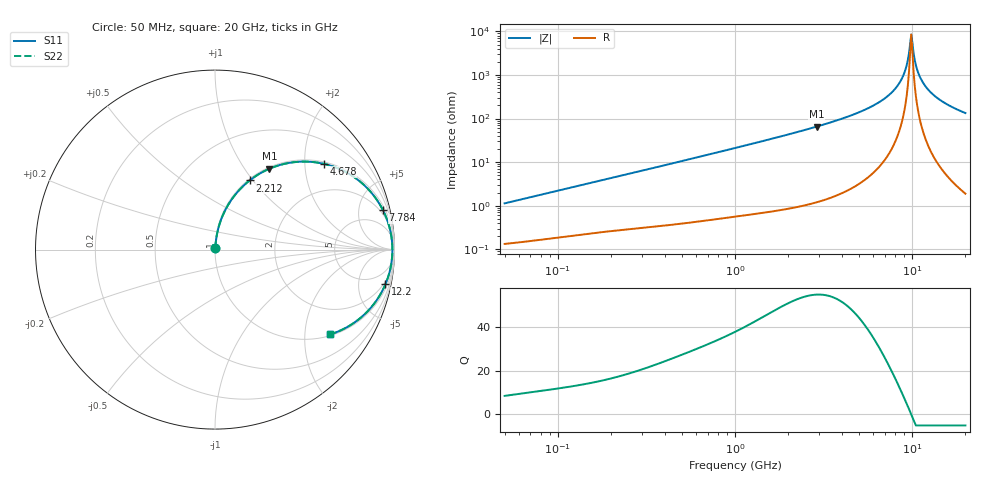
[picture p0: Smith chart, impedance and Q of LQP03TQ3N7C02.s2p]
!Murata Part Number: LQP03TQ3N7C02
!These Parameters are Measured in Series Mode Connection
!  o--[Z]--o
!Port1  Port2
!  o-------o
!Freq. Start=50[MHz] Stop=20[GHz], 401[Steps]
# Hz S RI R 50
!Freq.(Hz) S11(Real) S11(Imag) S21(Real) S21(Imag) S12(Real) S12(Imag) S22(Real) S22(Imag)
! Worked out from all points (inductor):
!   401 points, 50 MHz to 20 GHz, reference 50 ohm
!   read as one part in series: L = 3.55 nH near 51.52 MHz
!   highest Q = 54.6 at 2.896 GHz (marker M1), where L = 3.6 nH
!   self-resonance near 9.892 GHz
!   S11 on the Smith chart (normalised r, x): 50 MHz: 1.00, +0.02; 2.212 GHz: 1.02, +0.96; 4.678 GHz: 1.05, +2.49; 7.784 GHz: 1.45, +8.40; 12.2 GHz: 1.53, -9.67; 20 GHz: 1.04, -2.68
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5e7  0.00145 0.0112  0.9985 -0.0112  0.9985 -0.0112  0.00145 0.0112
1.364002e8  0.00305 0.0295  0.9969 -0.0295  0.9969 -0.0295  0.00305 0.0295
3.721004e8  0.0095 0.0778  0.9905 -0.0778  0.9905 -0.0778  0.0095 0.0778
1e9  0.0474 0.1995  0.9526 -0.1995  0.9526 -0.1995  0.0474 0.1995
2.211938e9  0.1932 0.3853  0.8068 -0.3853  0.8068 -0.3853  0.1932 0.3853
2.728004e9  0.2753 0.4376  0.7247 -0.4376  0.7247 -0.4376  0.2753 0.4376
2.896447e9  0.3036 0.4507  0.6964 -0.4507  0.6964 -0.4507  0.3036 0.4507
4.677679e9  0.6053 0.4782  0.3947 -0.4782  0.3947 -0.4782  0.6053 0.4782
6.125241e9  0.8007 0.3851  0.1993 -0.3851  0.1993 -0.3851  0.8007 0.3851
7.442007e9  0.9158 0.2557  0.0842 -0.2557  0.0842 -0.2557  0.9158 0.2557
7.784049e9  0.936 0.2194  0.064 -0.2194  0.064 -0.2194  0.936 0.2194
8.907419e9  0.9778 0.0999  0.0222 -0.0999  0.0222 -0.0999  0.9778 0.0999
9.316812e9  0.9848 0.0576  0.0152 -0.0576  0.0152 -0.0576  0.9848 0.0576
9.745021e9  0.9881 0.0149  0.0119 -0.0149  0.0119 -0.0149  0.9881 0.0149
9.892087e9  0.9884 0.000549  0.0116 -0.000549  0.0116 -0.000549  0.9884 0.000549
1.019291e10  0.9877 -0.0281  0.0123 0.0281  0.0123 0.0281  0.9877 -0.0281
1.050288e10  0.9853 -0.0566  0.0147 0.0566  0.0147 0.0566  0.9853 -0.0566
1.082228e10  0.9813 -0.0849  0.0187 0.0849  0.0187 0.0849  0.9813 -0.0849
1.131968e10  0.9723 -0.1267  0.0277 0.1267  0.0277 0.1267  0.9723 -0.1267
1.220001e10  0.9495 -0.1936  0.0505 0.1936  0.0505 0.1936  0.9495 -0.1936
1.504638e10  0.8424 -0.3517  0.1576 0.3517  0.1576 0.3517  0.8424 -0.3517
2e10  0.6401 -0.473  0.3599 0.473  0.3599 0.473  0.6401 -0.473
